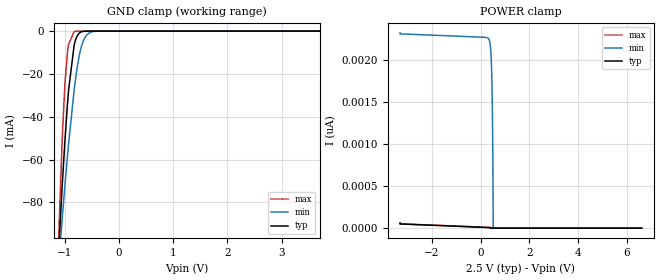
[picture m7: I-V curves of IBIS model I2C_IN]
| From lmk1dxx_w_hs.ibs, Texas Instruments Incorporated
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|   I2C_IN Model
[Model]   I2C_IN
Model_type   Input
Vinl = 0.75
Vinh = 1.75
|   typ   min   max
C_comp   1.91pF   1.79pF   2.03pF
[Voltage Range]   2.5   2.375   2.625
[Temperature Range]   45   150   -40
[Power Clamp Reference]   2.5   2.375   2.625
[GND Clamp Reference]   0   0   0
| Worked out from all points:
|   GND clamp passes 1 mA (typ) near -0.73 V on its own axis
[GND Clamp]
|   Voltage   I(typ)   I(min)   I(max)
-3.3V     -1.439A    -965.6mA   -2.519A
-1.104V   -99.75mA   -106.6mA   -92.35mA
-1.093V   -94.49mA   -103mA     -83.93mA
-1.046V   -72.46mA   -87.67mA   -50.92mA
-993.3mV  -50.39mA   -71.45mA   -23.74mA
-948.7mV  -34.17mA   -58.42mA   -9.928mA
-928mV    -27.6mA    -52.62mA   -6.14mA
-825mV    -6.529mA   -27.42mA   -189.4uA
-751.7mV  -1.581mA   -14.28mA   -14.66uA
-680.5mV  -245uA     -6.262mA   -5.632uA
-487.4mV  -5.258uA   -257.2uA   -4.934uA
6.6V      0A         0A         0A
[POWER Clamp]
|   Voltage   I(typ)   I(min)   I(max)
-3.3V     61.32pA    2.322nA    62.55pA
339.2mV   6.614pA    2.248nA    8.648pA
384.8mV   5.268pA    2.203nA    8.068pA
416.5mV   2.885pA    2.118nA    7.62pA
440.2mV   0A         1.987nA    7.192pA
457.1mV   0A         1.83nA     6.756pA
475.9mV   0A         1.548nA    5.964pA
491.7mV   0A         1.174nA    4.765pA
499.6mV   0A         920.4pA    3.832pA
507.5mV   0A         608.1pA    2.551pA
519.4mV   0A         0A         0A
6.6V      0A         0A         0A
